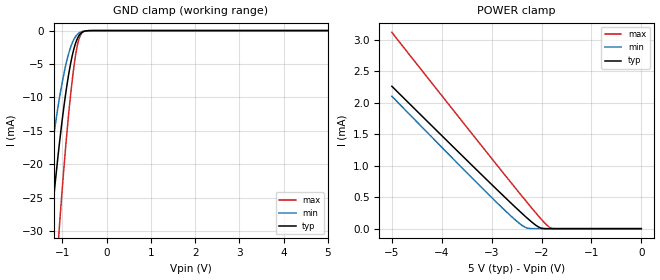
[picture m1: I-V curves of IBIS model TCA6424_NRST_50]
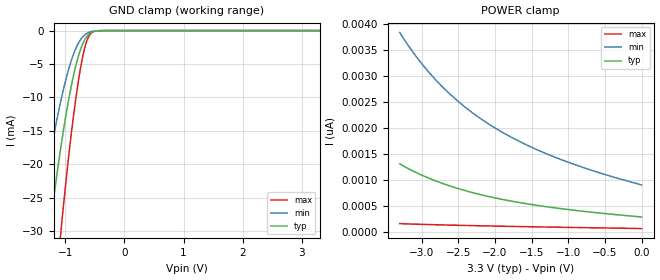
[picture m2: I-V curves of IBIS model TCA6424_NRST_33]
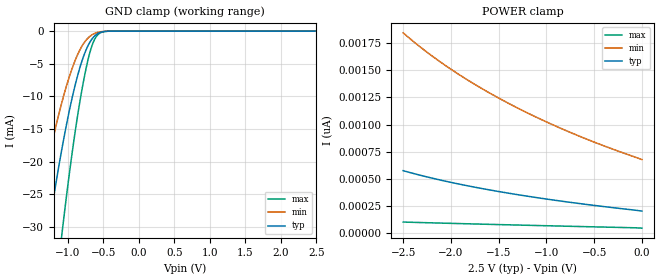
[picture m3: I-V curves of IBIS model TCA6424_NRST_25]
| TEXAS INSTRUMENTS INCORPORATED
| Standard Linear and Logic Group
| IBIS Model of TCA6424
| LOW-VOLTAGE 24-BIT I2C AND SMBus I/O EXPANDER WITH INTERRUPT OUTPUT,
| RESET, AND CONFIGURATION REGISTERS
| This file contains package information for the following:
|  QFN 32-pin (RGJ) package as [Component] TCA6424_RGJ
| This device can be powered at the following Vccs:
|  5 volt Vcc
|  3.3 volt Vcc
|  2.5 volt Vcc
|  1.8 volt Vcc
| This file provides unique models under the [Model Selector] for each Vcc.
| For operation at a specific Vcc, select the appropriate model after each
| [Model Selector] keyword.
[IBIS Ver]   3.2
[Comment char]  |_char
[File Name]   tca6424.ibs
[File Rev]   1.0 | x_die
[Date]   July 13, 2009
[Source]   Data created from TI-SPICE simulations at TI-SLL.
[Notes]   The following is an IBIS list for the TCA6424.
   Please contact sllibis@ti.com with questions and
   comments concerning SLL IBIS models.
[Disclaimer] Property of Texas Instruments Incorporated.  Unauthorized
   reproduction and/or distribution is strictly prohibited.
   This product is protected under copyright law.
   Created  2008, (C) Copyright  2008, Texas Instruments
   Incorporated, All Rights Reserved
   UNLESS THERE IS A SIGNED, WRITTEN AGREEMENT TO THE
   CONTRARY, TEXAS INSTRUMENTS (TI) IS PROVIDING THE IBIS
   MODELS  AND WITHOUT ANY WARRANTY, EXPRESSED OR
   IMPLIED.  TI assumes no liability for:
   1) the accuracy of the IBIS models provided to your
   company;
   2) the proper functioning of these IBIS Models in your
   design or for any resulting applications; or
   3) infringement of patents, copyrights or intellectual
   property rights resulting from your use of these IBIS
   models.
   TI provides IBIS Models as a service to our customers.
   You and your company shall not distribute, sell or give
   these models to anyone else without prior written
   permission from TI.
   TI reserves the right to make changes to our products or
   to discontinue any semiconductor product or service
   without notice, and advises our customers to obtain the
   latest version of relevant information to verify, before
   placing orders, that the information being relied on is
   current.
   Please be aware that your receipt and use of the IBIS
   information provided shall serve as acceptance of these
   terms and conditions.  If you do not accept these terms,
   you should return or destroy the IBIS models and any
   other accompanying information immediately.
| Component TCA6424_RGJ 32-PIN QFN
[Component]   TCA6424_PW
[Manufacturer]   Texas Instruments, Inc.
[Package]
|   typ   min   max
R_pkg   4.500e-02   3.800e-02   5.100e-02
L_pkg   2.593e-09   2.447e-09   3.080e-09
C_pkg   2.810e-13   2.430e-13   3.770e-13
[Pin]   signal_name   model_name   R_pin   L_pin   C_pin
1   P00   TCA6424_P   5.100e-02   2.447e-09   2.430e-13
2   P01   TCA6424_P   5.100e-02   2.447e-09   2.430e-13
3   P02   TCA6424_P   5.100e-02   2.512e-09   2.550e-13
4   P03   TCA6424_P   3.800e-02   2.458e-09   2.810e-13
5   P04   TCA6424_P   3.900e-02   2.832e-09   3.160e-13
6   P05   TCA6424_P   3.800e-02   2.460e-09   2.790e-13
7   P06   TCA6424_P   5.100e-02   2.512e-09   2.550e-13
8   P07   TCA6424_P   5.100e-02   2.447e-09   2.430e-13
9   P10   TCA6424_P   5.100e-02   2.447e-09   2.430e-13
10   P11   TCA6424_P   5.100e-02   2.447e-09   2.430e-13
11   P12   TCA6424_P   5.100e-02   2.512e-09   2.550e-13
12   P13   TCA6424_P   3.800e-02   2.458e-09   2.810e-13
13   P14   TCA6424_P   3.900e-02   2.832e-09   3.160e-13
14   P15   TCA6424_P   3.800e-02   2.460e-09   2.790e-13
15   P16   TCA6424_P   5.100e-02   2.512e-09   2.550e-13
16   P17   TCA6424_P   5.100e-02   2.447e-09   2.430e-13
17   P20   TCA6424_P   5.100e-02   2.447e-09   2.430e-13
18   P21   TCA6424_P   5.100e-02   2.447e-09   2.430e-13
19   P22   TCA6424_P   5.100e-02   2.512e-09   2.550e-13
20   P23   TCA6424_P   3.800e-02   2.458e-09   2.810e-13
21   P24   TCA6424_P   3.900e-02   2.832e-09   3.160e-13
22   P25   TCA6424_P   3.800e-02   2.460e-09   2.790e-13
23   P26   TCA6424_P   5.100e-02   2.512e-09   2.550e-13
24   P27   TCA6424_P   5.100e-02   2.447e-09   2.430e-13
25   GND   GND   4.000e-02   3.080e-09   3.770e-13
26   ADDR   TCA6424_ADDR   3.800e-02   2.458e-09   2.810e-13
27   VCCP   POWER   3.900e-02   2.832e-09   3.160e-13
28   NRESET   TCA6424_NRST   5.100e-02   2.512e-09   2.550e-13
29   SCL   TCA6424_SCL   5.100e-02   2.512e-09   2.550e-13
30   SDA   TCA6424_SDA   3.800e-02   2.459e-09   2.790e-13
31   VCCI   POWER   4.000e-02   3.080e-09   3.770e-13
32   NINT   TCA6424_NINT   5.100e-02   2.447e-09   2.430e-13
| Model TCA6424_NRST
[Model Selector]   TCA6424_NRST
TCA6424_NRST_50   5 volt Vcc
TCA6424_NRST_33   3.3 volt Vcc
TCA6424_NRST_25   2.5 volt Vcc
TCA6424_NRST_18   1.8 volt Vcc
| Model TCA6424_SCL
[Model Selector]   TCA6424_SCL
TCA6424_SCL_50   5 volt Vcc
TCA6424_SCL_33   3.3 volt Vcc
TCA6424_SCL_25   2.5 volt Vcc
TCA6424_SCL_18   1.8 volt Vcc
| Model TCA6424_ADDR
[Model Selector]   TCA6424_ADDR
TCA6424_ADDR_50   5 volt Vcc
TCA6424_ADDR_33   3.3 volt Vcc
TCA6424_ADDR_25   2.5 volt Vcc
TCA6424_ADDR_18   1.8 volt Vcc
| Model TCA6424_P
[Model Selector]   TCA6424_P
TCA6424_P_50   5 volt Vcc
TCA6424_P_33   3.3 volt Vcc
TCA6424_P_25   2.5 volt Vcc
TCA6424_P_18   1.8 volt Vcc
| Model TCA6424_SDA
[Model Selector]   TCA6424_SDA
TCA6424_SDA_50   5 volt Vcc
TCA6424_SDA_33   3.3 volt Vcc
TCA6424_SDA_25   2.5 volt Vcc
TCA6424_SDA_18   1.8 volt Vcc
| Model TCA6424_NINT
[Model Selector]   TCA6424_NINT
TCA6424_NINT_50   5 volt Vcc
TCA6424_NINT_33   3.3 volt Vcc
TCA6424_NINT_25   2.5 volt Vcc
TCA6424_NINT_18   1.8 volt Vcc
| Models and submodels in the file (24): TCA6424_NRST_50 (Input), TCA6424_NRST_33 (Input), TCA6424_NRST_25 (Input), TCA6424_NRST_18 (Input), TCA6424_SCL_50 (Input), TCA6424_SCL_33 (Input), TCA6424_SCL_25 (Input), TCA6424_SCL_18 (Input), TCA6424_ADDR_50 (Input), TCA6424_ADDR_33 (Input), TCA6424_ADDR_25 (Input), TCA6424_ADDR_18 (Input), TCA6424_P_50 (I/O), TCA6424_P_33 (I/O), TCA6424_P_25 (I/O), TCA6424_P_18 (I/O), TCA6424_SDA_50 (I/O_open_drain), TCA6424_SDA_33 (I/O_open_drain), TCA6424_SDA_25 (I/O_open_drain), TCA6424_SDA_18 (I/O_open_drain), TCA6424_NINT_50 (Open_drain), TCA6424_NINT_33 (Open_drain), TCA6424_NINT_25 (Open_drain), TCA6424_NINT_18 (Open_drain)
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[Model]   TCA6424_NRST_50
Model_type  Input
Vinl=1.35
Vinh=3.85
| variable   typ   min   max
C_comp   2.17pF   1.80pF   2.32pF
[Temperature Range]   40   100   -40
| Ambient temperature   25   85   -40
[Voltage range]   5   4.5   5.5
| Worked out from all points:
|   GND clamp passes 1 mA (typ) near -0.65 V on its own axis
|   POWER clamp passes 1 mA (typ) near -3.39 V on its own axis
[GND Clamp]
| TCA6424_NRST_50
|   Voltage   I(typ)   I(min)   I(max)
-5V       -421.5mA   -327.2mA   -555.2mA
-1.48V    -46.19mA   -30.98mA   -72.79mA
-1.435V   -42.57mA   -28.34mA   -67.61mA
-1.265V   -29.76mA   -19.1mA    -48.89mA
-1.085V   -17.96mA   -10.85mA   -30.98mA
-1.065V   -16.78mA   -10.05mA   -29.14mA
-930mV    -9.662mA   -5.357mA   -17.73mA
-795mV    -4.307mA   -2.154mA   -8.462mA
-680mV    -1.498mA   -708.4uA   -2.836mA
-585mV    -416.3uA   -213.5uA   -615.5uA
-405mV    -11.9uA    -9.596uA   -9.604uA
5V        572.5pA    2.003nA    91.86pA
[POWER Clamp]
| TCA6424_NRST_50
|   Voltage   I(typ)   I(min)   I(max)
-5V       2.259mA    2.101mA    3.114mA
-3.24V    886.3uA    684.1uA    1.353mA
-2.49V    314.9uA    114.8uA    611.7uA
-2.3V     176.9uA    14.07uA    427.1uA
-2.08V    36.49uA    30.1nA     218.5uA
-1.99V    5.536uA    5.854nA    137uA
-1.86V    59.38nA    4.002nA    34.02uA
-1.805V   9.042nA    3.854nA    7.955uA
-1.735V   1.991nA    3.696nA    355.1nA
-84.45fV  572.5pA    1.628nA    108.3pA
[Model]   TCA6424_NRST_33
Model_type  Input
Vinl=0.9
Vinh=2.52
| variable   typ   min   max
C_comp   2.22pF   1.76pF   2.42pF
[Temperature Range]   40   100   -40
| Ambient temperature   25   85   -40
[Voltage range]   3.3   3   3.6
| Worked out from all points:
|   GND clamp passes 1 mA (typ) near -0.65 V on its own axis
[GND Clamp]
| TCA6424_NRST_33
|   Voltage   I(typ)   I(min)   I(max)
-3.3V     -229.8mA   -173.1mA   -314.8mA
-1.49V    -47mA      -31.57mA   -73.96mA
-1.455V   -44.17mA   -29.5mA    -69.9mA
-1.285V   -31.19mA   -20.13mA   -51.01mA
-1.255V   -29.05mA   -18.6mA    -47.84mA
-1.08V    -17.66mA   -10.65mA   -30.52mA
-945mV    -10.37mA   -5.81mA    -18.9mA
-810mV    -4.799mA   -2.428mA   -9.366mA
-700mV    -1.861mA   -882.4uA   -3.61mA
-615mV    -655uA     -320.4uA   -1.07mA
-410mV    -13.36uA   -10.66uA   -11.01uA
3.3V      289.3pA    1.025nA    57.78pA
[POWER Clamp]
| TCA6424_NRST_33
|   Voltage   I(typ)   I(min)   I(max)
-3.3V     1.315nA    3.842nA    162.7pA
-3.18V    1.219nA    3.582nA    157.1pA
-3.035V   1.119nA    3.303nA    150.7pA
-2.89V    1.03nA     3.055nA    144.8pA
-2.74V    948.5pA    2.827nA    139.1pA
-2.585V   873.6pA    2.616nA    133.6pA
-2.42V    803.1pA    2.417nA    128.2pA
-2.06V    676pA      2.056nA    117.3pA
-1.65V    564.5pA    1.732nA    106.3pA
-1.18V    465.7pA    1.439nA    94.89pA
-640mV    376.5pA    1.169nA    82.73pA
-48.03fV  289.3pA    907.3pA    66.29pA
[Model]   TCA6424_NRST_25
Model_type  Input
Vinl=0.69
Vinh=1.89
| variable   typ   min   max
C_comp   2.23pF   1.74pF   2.48pF
[Temperature Range]   40   100   -40
| Ambient temperature   25   85   -40
[Voltage range]   2.5   2.3   2.7
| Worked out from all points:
|   GND clamp passes 1 mA (typ) near -0.65 V on its own axis
[GND Clamp]
| TCA6424_NRST_25
|   Voltage   I(typ)   I(min)   I(max)
-2.5V     -143.4mA   -105mA     -204.1mA
-1.49V    -47mA      -31.57mA   -73.96mA
-1.46V    -44.57mA   -29.79mA   -70.48mA
-1.27V    -30.12mA   -19.36mA   -49.42mA
-1.085V   -17.96mA   -10.85mA   -30.98mA
-955mV    -10.86mA   -6.122mA   -19.7mA
-840mV    -5.866mA   -3.039mA   -11.27mA
-730mV    -2.504mA   -1.201mA   -4.956mA
-650mV    -1.048mA   -498.6uA   -1.878mA
-575mV    -354.2uA   -185.5uA   -505.4uA
-445mV    -29.23uA   -21.62uA   -27.21uA
2.5V      205.9pA    741.4pA    43.26pA
[POWER Clamp]
| TCA6424_NRST_25
|   Voltage   I(typ)   I(min)   I(max)
-2.5V     576.6pA    1.842nA    105.1pA
-2.26V    521.5pA    1.671nA    99.15pA
-2.005V   470.3pA    1.511nA    93.15pA
-1.725V   421pA      1.356nA    86.8pA
-1.425V   374.2pA    1.208nA    80.23pA
-1.1V     329.2pA    1.066nA    73.31pA
-760mV    287.2pA    932pA      66.26pA
-415mV    248.9pA    810.6pA    59.25pA
-31.15fV  205.9pA    679.1pA    48.93pA
